| IBIS file for GS8662xxxBD
| Package: standard 165pin BGA
| DQ driver is programmable
| VDD 1.8V, VDDQ 1.5V or 1.8V
| Date:
| Rev 1.1 11/12/10 1) Pin F10 on Q36 pacakge changed from DIN to PROGBUF
[IBIS Ver]   4.2
[File name]   8662xxxbd.ibs
[File Rev]   1.1
[Date]   11/12/10
[Component]   GS8662D08BD
[Manufacturer]   GSI Technology
[Package]
|  variable   typ   min   max
R_pkg   0.2   0.1   0.5
L_pkg   3nH   1nH   5nH
C_pkg   1.5pF   1pF   3pF
[Package Model]   8662xxxBD
[Pin Mapping] pulldown_ref pullup_ref gnd_clamp_ref power_clamp_ref ext_ref
|PIN   Pull-Down   Pull-Up   Power-clamp   Gnd-clamp   EXT-ref
 A1   VSS   VDDQ   VSS   VDD
 A2   NC   NC   VSS   VDD   VREF
 A3   NC   NC   VSS   VDD   VREF
 A4   NC   NC   VSS   VDD   VREF
 A5   NC   NC   VSS   VDD   VREF
 A6   NC   NC   VSS   VDD   VREF
 A7   NC   NC   VSS   VDD   VREF
 A8   NC   NC   VSS   VDD   VREF
 A9   NC   NC   VSS   VDD   VREF
 A10   NC   NC   VSS   VDD   VREF
 A11   VSS   VDDQ   VSS   VDD
 B1   NC   NC
 B2   NC   NC
 B3   NC   NC
 B4   NC   NC   VSS   VDD   VREF
 B5   NC   NC
 B6   NC   NC   VSS   VDD   VREF
 B7   NC   NC   VSS   VDD   VREF
 B8   NC   NC   VSS   VDD   VREF
 B9   NC   NC
 B10   NC   NC
 B11   VSS   VDDQ   VSS   VDD
 C1   NC   NC
 C2   NC   NC
 C3   NC   NC
 C4   VSS   NC
 C5   NC   NC   VSS   VDD   VREF
 C6   NC   NC
 C7   NC   NC   VSS   VDD   VREF
 C8   VSS   NC
 C9   NC   NC
C10   NC   NC
 C11   NC   NC   VSS   VDD   VREF
 D1   NC   NC
 D2   NC   NC   VSS   VDD   VREF
 D3   NC   NC
 D4   VSS   NC
 D5   VSS   NC
 D6   VSS   NC
 D7   VSS   NC
 D8   VSS   NC
 D9   NC   NC
 D10   NC   NC
 D11   NC   NC
 E1   NC   NC
 E2   NC   NC
 E3   NC   NC
 E4   NC   VDDQ
 E5   VSS   NC
 E6   VSS   NC
 E7   VSS   NC
 E8   NC   VDDQ
 E9   NC   NC
 E10   NC   NC   VSS   VDD   VREF
 E11   VSS   VDDQ   VSS   VDD
 F1   NC   NC
 F2   NC   NC
 F3   NC   NC
 F4   NC   VDDQ
 F5   NC   VDD
 F6   VSS   NC
 F7   NC   VDD
 F8   NC   VDDQ
 F9   NC   NC
 F10   NC   NC
 F11   NC   NC
 G1   NC   NC
 G2   NC   NC   VSS   VDD   VREF
 G3   VSS   VDDQ   VSS   VDD
 G4   NC   VDDQ
 G5   NC   VDD
 G6   VSS   NC
 G7   NC   VDD
 G8   NC   VDDQ
 G9   NC   NC
 G10   NC   NC
 G11   NC   NC
 H1   NC   NC   VSS   VDD   VREF
 H2   NC   VREF
 H3   NC   VDDQ
 H4   NC   VDDQ
 H5   NC   VDD
 H6   VSS   NC
 H7   NC   VDD
 H8   NC   VDDQ
 H9   NC   VDDQ
 H10   NC   VREF
 H11   NC   NC
 J1   NC   NC
 J2   NC   NC
 J3   NC   NC
 J4   NC   VDDQ
 J5   NC   VDD
 J6   VSS   NC
 J7   NC   VDD
 J8   NC   VDDQ
 J9   NC   NC
 J10   VSS   VDDQ   VSS   VDD
 J11   NC   NC   VSS   VDD   VREF
 K1   NC   NC
 K2   NC   NC
 K3   NC   NC
 K4   NC   VDDQ
 K5   NC   VDD
 K6   VSS   NC
 K7   NC   VDD
 K8   NC   VDDQ
 K9   NC   NC
 K10   NC   NC
 K11   NC   NC
 L1   NC   NC
 L2   VSS   VDDQ   VSS   VDD
 L3   NC   NC   VSS   VDD   VREF
 L4   NC   VDDQ
 L5   VSS   NC
 L6   VSS   NC
 L7   VSS   NC
 L8   NC   VDDQ
 L9   NC   NC
 L10   NC   NC
 L11   VSS   VDDQ   VSS   VDD
 M1   NC   NC
 M2   NC   NC
 M3   NC   NC
 M4   VSS   NC
 M5   VSS   NC
 M6   VSS   NC
 M7   VSS   NC
 M8   VSS   NC
 M9   NC   NC
 M10   NC   NC
 M11   NC   NC   VSS   VDD   VREF
 N1   NC   NC
 N2   NC   NC   VSS   VDD   VREF
 N3   NC   NC
 N4   VSS   NC
 N5   NC   NC   VSS   VDD   VREF
 N6   NC   NC   VSS   VDD   VREF
 N7   NC   NC   VSS   VDD   VREF
 N8   VSS   NC
 N9   NC   NC
 N10   NC   NC
 N11   NC   NC
 P1   NC   NC
 P2   NC   NC
 P3   VSS   VDDQ   VSS   VDD
 P4   NC   NC   VSS   VDD   VREF
 P5   NC   NC   VSS   VDD   VREF
 P6   NC   NC   VSS   VDD   VREF
 P7   NC   NC   VSS   VDD   VREF
 P8   NC   NC   VSS   VDD   VREF
 P9   NC   NC
 P10   NC   NC
 P11   NC   NC
 R1   VSS   VDDQ   VSS   VDD
 R2   NC   NC   VSS   VDD   VREF
 R3   NC   NC   VSS   VDD   VREF
 R4   NC   NC   VSS   VDD   VREF
 R5   NC   NC   VSS   VDD   VREF
 R6   NC   NC   VSS   VDD   VREF
 R7   NC   NC   VSS   VDD   VREF
 R8   NC   NC   VSS   VDD   VREF
 R9   NC   NC   VSS   VDD   VREF
 R10   NC   NC   VSS   VDD   VREF
 R11   NC   NC   VSS   VDD   VREF
[Pin]   signal_name model_name   R_pin   L_pin   C_pin
 A1   nCQ   ECHO   229m   1.82nH   0.656pF
 A2   SA   CONTROL   203m   1.74nH   0.634pF
 A3   SA   CONTROL   185m   1.59nH   0.518pF
 A4   nW   CONTROL   185m   1.38nH   0.583pF
 A5   nNW1   CONTROL   178m   1.36nH   0.540pF
 A6   nK   CONTROL   224m   1.64nH   0.652pF
 A7   SA   CONTROL   185m   1.39nH   0.547pF
 A8   nR   CONTROL   188m   1.49nH   0.551pF
 A9   SA   CONTROL   186m   1.48nH   0.595pF
 A10   SA   CONTROL   191m   1.70nH   0.568pF
 A11   CQ   ECHO   227m   1.84nH   0.605pF
 B1   NC   NC
 B2   NC   NC
 B3   NC   NC
 B4   SA   CONTROL   181m   1.49nH   0.521pF
 B5   NC   NC
 B6   K   CONTROL   221m   1.68nH   0.652pF
 B7   nNW0   CONTROL   178m   1.43nH   0.537pF
 B8   SA   CONTROL   181m   1.41nH   0.565pF
 B9   NC   NC
 B10   NC   NC
 B11   Q3   PROGBUF   232m   1.94nH   0.683pF
 C1   NC   NC
 C2   NC   NC
 C3   NC   NC
 C4   VSS   GND
 C5   SA   CONTROL   189m   1.61nH   0.614pF
 C6   NC   NC
 C7   SA   CONTROL   185m   1.72nH   0.535pF
 C8   VSS   GND
 C9   NC   NC
 C10   NC   NC
 C11   D3   DIN   219m   1.74nH   0.625pF
 D1   NC   NC
 D2   D4   DIN   227m   1.95nH   0.654pF
 D3   NC   NC
 D4   VSS   GND
 D5   VSS   GND
 D6   VSS   GND
 D7   VSS   GND
 D8   VSS   GND
 D9   NC   NC
 D10   NC   NC
 D11   Nc   NC
 E1   Nc   NC
 E2   Nc   NC
 E3   Q4   PROGBUF   240m   2.04nH   0.712pF
 E4   VDDQ   POWER
 E5   VSS   GND
 E6   VSS   GND
 E7   VSS   GND
 E8   VDDQ   POWER
 E9   NC   NC
 E10   D2   DIN   223m   1.85nH   0.659pF
 E11   Q2   PROGBUF   225m   1.74nH   0.649pF
 F1   NC   NC
 F2   NC   NC
 F3   NC   NC
 F4   VDDQ   POWER
 F5   VDD   POWER
 F6   VSS   GND
 F7   VDD   POWER
 F8   VDDQ   POWER
 F9   NC   NC
 F10   NC   NC
 F11   NC   NC
 G1   NC   NC
 G2   D5   DIN   221m   1.73nH   0.669pF
 G3   Q5   PROGBUF   244m   2.11nH   0.723pF
 G4   VDDQ   POWER
 G5   VDD   POWER
 G6   VSS   GND
 G7   VDD   POWER
 G8   VDDQ   POWER
 G9   NC   NC
 G10   NC   NC
 G11   NC   NC
 H1   NDoff   CONTROL   254m   2.26nH   0.651pF
 H2   VREF   POWER
 H3   VDDQ   POWER
 H4   VDDQ   POWER
 H5   VDD   POWER
 H6   VSS   GND
 H7   VDD   POWER
 H8   VDDQ   POWER
 H9   VDDQ   POWER
 H10   VREF   POWER
 H11   ZQ   NC
 J1   NC   NC
 J2   NC   NC
 J3   NC   NC
 J4   VDDQ   POWER
 J5   VDD   POWER
 J6   VSS   GND
 J7   VDD   POWER
 J8   VDDQ   POWER
 J9   NC   NC
 J10   Q1   PROGBUF   231m   1.92nH   0.628pF
 J11   D1   DIN   222m   1.68nH   0.657pF
 K1   NC   NC
 K2   NC   NC
 K3   NC   NC
 K4   VDDQ   POWER
 K5   VDD   POWER
 K6   VSS   GND
 K7   VDD   POWER
 K8   VDDQ   POWER
 K9   NC   NC
 K10   NC   NC
 K11   NC   NC
 L1   NC   NC
 L2   Q6   PROGBUF   228m   1.89nH   0.672pF
 L3   D6   DIN   237m   2.14nH   0.663pF
 L4   VDDQ   POWER
 L5   VSS   GND
 L6   VSS   GND
 L7   VSS   GND
 L8   VDDQ   POWER
 L9   NC   NC
 L10   NC   NC
 L11   Q0   PROGBUF   223m   1.72nH   0.654pF
 M1   NC   NC
 M2   NC   NC
 M3   NC   NC
 M4   VSS   GND
 M5   VSS   GND
 M6   VSS   GND
 M7   VSS   GND
 M8   VSS   GND
 M9   NC   NC
 M10   NC   NC
 M11   D0   DIN   228m   1.90nH   0.609pF
 N1   NC   NC
 N2   D7   DIN   219m   1.88nH   0.569pF
 N3   NC   NC
 N4   VSS   GND
 N5   SA   CONTROL   186m   1.69nH   0.505pF
 N6   SA   CONTROL   191m   1.56nH   0.607pF
 N7   SA   CONTROL   193m   1.62nH   0.543pF
 N8   VSS   GND
 N9   NC   NC
 N10   NC   NC
 N11   NC   NC
 P1   NC   NC
 P2   NC   NC
 P3   Q7   PROGBUF   236m   2.33nH   0.676pF
 P4   SA   CONTROL   185m   1.52nH   0.546pF
 P5   SA   CONTROL   185m   1.41nH   0.604pF
 P6   C   CONTROL   184m   1.42nH   0.590pF
 P7   SA   CONTROL   192m   1.57nH   0.599pF
 P8   SA   CONTROL   195m   1.51nH   0.593pF
 P9   NC   NC
 P10   NC   NC
 P11   NC   NC
 R1   TDO   JTAG   151m   1.27nH   0.509pF
 R2   TCK   CONTROL   132m   1.10nH   0.478pF
 R3   SA   CONTROL   208m   1.92nH   0.490pF
 R4   SA   CONTROL   198m   1.58nH   0.599pF
 R5   SA   CONTROL   190m   1.46nH   0.609pF
 R6   CBar   CONTROL   196m   1.46nH   0.608pF
 R7   SA   CONTROL   198m   1.47nH   0.632pF
 R8   SA   CONTROL   202m   1.49nH   0.640pF
 R9   SA   CONTROL   214m   1.68nH   0.647pF
 R10   TMS   CONTROL   148m   1.19nH   0.517pF
 R11   TDI   CONTROL   157m   1.27nH   0.525pF
[Component]   GS8662D09BD
[Manufacturer]   GSI Technology
[Package]
|  variable   typ   min   max
R_pkg   0.2   0.1   0.5
L_pkg   3nH   1nH   5nH
C_pkg   1.5pF   1pF   3pF
[Package Model]   8662xxxBD
[Pin Mapping] pulldown_ref pullup_ref gnd_clamp_ref power_clamp_ref ext_ref
|PIN   Pull-Down   Pull-Up   Power-clamp   Gnd-clamp   EXT-ref
 A1   VSS   VDDQ   VSS   VDD
 A2   NC   NC   VSS   VDD   VREF
 A3   NC   NC   VSS   VDD   VREF
 A4   NC   NC   VSS   VDD   VREF
 A5   NC   NC   VSS   VDD   VREF
 A6   NC   NC   VSS   VDD   VREF
 A7   NC   NC   VSS   VDD   VREF
 A8   NC   NC   VSS   VDD   VREF
 A9   NC   NC   VSS   VDD   VREF
 A10   NC   NC   VSS   VDD   VREF
 A11   VSS   VDDQ   VSS   VDD
 B1   NC   NC
 B2   NC   NC
 B3   NC   NC
 B4   NC   NC   VSS   VDD   VREF
 B5   NC   NC
 B6   NC   NC   VSS   VDD   VREF
 B7   NC   NC   VSS   VDD   VREF
 B8   NC   NC   VSS   VDD   VREF
 B9   NC   NC
 B10   NC   NC
 B11   VSS   VDDQ   VSS   VDD
 C1   NC   NC
 C2   NC   NC
 C3   NC   NC
 C4   VSS   NC
 C5   NC   NC   VSS   VDD   VREF
 C6   NC   NC
 C7   NC   NC   VSS   VDD   VREF
 C8   VSS   NC
 C9   NC   NC
 C10   NC   NC
 C11   NC   NC   VSS   VDD   VREF
 D1   NC   NC
 D2   NC   NC   VSS   VDD   VREF
 D3   NC   NC
 D4   VSS   NC
 D5   VSS   NC
 D6   VSS   NC
 D7   VSS   NC
 D8   VSS   NC
 D9   NC   NC
 D10   NC   NC
 D11   NC   NC
 E1   NC   NC
 E2   NC   NC
 E3   VSS   VDDQ   VSS   VDD
 E4   NC   VDDQ
 E5   VSS   NC
 E6   VSS   NC
 E7   VSS   NC
 E8   NC   VDDQ
 E9   NC   NC
 E10   NC   NC   VSS   VDD   VREF
 E11   VSS   VDDQ   VSS   VDD
 F1   NC   NC
 F2   NC   NC
 F3   NC   NC
 F4   NC   VDDQ
 F5   NC   VDD
 F6   VSS   NC
 F7   NC   VDD
 F8   NC   VDDQ
 F9   NC   NC
 F10   NC   NC
 F11   NC   NC
 G1   NC   NC
 G2   NC   NC   VSS   VDD   VREF
 G3   VSS   VDDQ   VSS   VDD
 G4   NC   VDDQ
 G5   NC   VDD
 G6   VSS   NC
 G7   NC   VDD
 G8   NC   VDDQ
 G9   NC   NC
 G10   NC   NC
 G11   NC   NC
 H1   NC   NC   VSS   VDD   VREF
 H2   NC   VREF
 H3   NC   VDDQ
 H4   NC   VDDQ
 H5   NC   VDD
 H6   VSS   NC
 H7   NC   VDD
 H8   NC   VDDQ
 H9   NC   VDDQ
 H10   NC   VREF
 H11   NC   NC
 J1   NC   NC
 J2   NC   NC
 J3   NC   NC
 J4   NC   VDDQ
 J5   NC   VDD
 J6   VSS   NC
 J7   NC   VDD
 J8   NC   VDDQ
 J9   NC   NC
 J10   VSS   VDDQ   VSS   VDD
 J11   NC   NC   VSS   VDD   VREF
 K1   NC   NC
 K2   NC   NC
 K3   NC   NC
 K4   NC   VDDQ
 K5   NC   VDD
 K6   VSS   NC
 K7   NC   VDD
 K8   NC   VDDQ
 K9   NC   NC
 K10   NC   NC
 K11   NC   NC
 L1   NC   NC
 L2   VSS   VDDQ   VSS   VDD
 L3   NC   NC   VSS   VDD   VREF
 L4   NC   VDDQ
 L5   VSS   NC
 L6   VSS   NC
 L7   VSS   NC
 L8   NC   VDDQ
 L9   NC   NC
 L10   NC   NC
 L11   VSS   VDDQ   VSS   VDD
 M1   NC   NC
 M2   NC   NC
 M3   NC   NC
 M4   VSS   NC
 M5   VSS   NC
 M6   VSS   NC
 M7   VSS   NC
 M8   VSS   NC
 M9   NC   NC
 M10   NC   NC
 M11   NC   NC   VSS   VDD   VREF
 N1   NC   NC
 N2   NC   NC   VSS   VDD   VREF
 N3   NC   NC
 N4   VSS   NC
 N5   NC   NC   VSS   VDD   VREF
 N6   NC   NC   VSS   VDD   VREF
 N7   NC   NC   VSS   VDD   VREF
 N8   VSS   NC
 N9   NC   NC
 N10   NC   NC
 N11   NC   NC
 P1   NC   NC
 P2   NC   NC
 P3   VSS   VDDQ   VSS   VDD
 P4   NC   NC   VSS   VDD   VREF
 P5   NC   NC   VSS   VDD   VREF
 P6   NC   NC   VSS   VDD   VREF
 P7   NC   NC   VSS   VDD   VREF
 P8   NC   NC   VSS   VDD   VREF
 P9   NC   NC
 P10   NC   NC   VSS   VDD   VREF
 P11   VSS   VDDQ   VSS   VDD
 R1   VSS   VDDQ   VSS   VDD
 R2   NC   NC   VSS   VDD   VREF
 R3   NC   NC   VSS   VDD   VREF
 R4   NC   NC   VSS   VDD   VREF
 R5   NC   NC   VSS   VDD   VREF
 R6   NC   NC   VSS   VDD   VREF
 R7   NC   NC   VSS   VDD   VREF
 R8   NC   NC   VSS   VDD   VREF
 R9   NC   NC   VSS   VDD   VREF
 R10   NC   NC   VSS   VDD   VREF
 R11   NC   NC   VSS   VDD   VREF
[Pin]   signal_name model_name   R_pin   L_pin   C_pin
 A1   nCQ   ECHO   229m   1.82nH   0.656pF
 A2   SA   CONTROL   203m   1.74nH   0.634pF
 A3   SA   CONTROL   185m   1.59nH   0.518pF
 A4   nW   CONTROL   185m   1.38nH   0.583pF
 A5   nBW1   CONTROL   178m   1.36nH   0.540pF
 A6   nK   CONTROL   224m   1.64nH   0.652pF
 A7   SA   CONTROL   185m   1.39nH   0.547pF
 A8   nR   CONTROL   188m   1.49nH   0.551pF
 A9   SA   CONTROL   186m   1.48nH   0.595pF
 A10   SA   CONTROL   191m   1.70nH   0.568pF
 A11   CQ   ECHO   227m   1.84nH   0.605pF
 B1   NC   NC
 B2   NC   NC
 B3   NC   NC
 B4   SA   CONTROL   181m   1.49nH   0.521pF
 B5   NC   NC
 B6   K   CONTROL   221m   1.68nH   0.652pF
 B7   NBW0   CONTROL   178m   1.43nH   0.537pF
 B8   SA   CONTROL   181m   1.41nH   0.565pF
 B9   NC   NC
 B10   NC   NC
 B11   Q4   PROGBUF   232m   1.94nH   0.683pF
 C1   NC   NC
 C2   NC   NC
 C3   NC   NC
 C4   VSS   GND
 C5   SA   CONTROL   189m   1.61nH   0.614pF
 C6   NC   NC
 C7   SA   CONTROL   185m   1.72nH   0.535pF
 C8   VSS   GND
 C9   NC   NC
 C10   NC   NC
 C11   D4   DIN   219m   1.74nH   0.625pF
 D1   NC   NC
 D2   D5   DIN   227m   1.95nH   0.654pF
 D3   NC   NC
 D4   VSS   GND
 D5   VSS   GND
 D6   VSS   GND
 D7   VSS   GND
 D8   VSS   GND
 D9   NC   NC
 D10   NC   NC
 D11   NC   NC
 E1   NC   NC
 E2   NC   NC
 E3   Q5   PROGBUF   240m   2.04nH   0.712pF
 E4   VDDQ   POWER
 E5   VSS   GND
 E6   VSS   GND
 E7   VSS   GND
 E8   VDDQ   POWER
 E9   NC   NC
 E10   D3   DIN   223m   1.85nH   0.659pF
 E11   Q3   PROGBUF   225m   1.74nH   0.649pF
 F1   NC   NC
 F2   NC   NC
 F3   NC   NC
 F4   VDDQ   POWER
 F5   VDD   POWER
 F6   VSS   GND
 F7   VDD   POWER
 F8   VDDQ   POWER
 F9   NC   NC
 F10   NC   NC
 F11   NC   NC
 G1   NC   NC
 G2   D6   DIN   221m   1.73nH   0.669pF
 G3   Q6   PROGBUF   244m   2.11nH   0.723pF
 G4   VDDQ   POWER
 G5   VDD   POWER
 G6   VSS   GND
 G7   VDD   POWER
 G8   VDDQ   POWER
 G9   NC   NC
 G10   NC   NC
 G11   NC   NC
 H1   NDoff   CONTROL   254m   2.26nH   0.651pF
 H2   VREF   POWER
 H3   VDDQ   POWER
 H4   VDDQ   POWER
 H5   VDD   POWER
 H6   VSS   GND
 H7   VDD   POWER
 H8   VDDQ   POWER
 H9   VDDQ   POWER
 H10   VREF   POWER
 H11   ZQ   NC
 J1   NC   NC
 J2   NC   NC
 J3   NC   NC
 J4   VDDQ   POWER
 J5   VDD   POWER
 J6   VSS   GND
 J7   VDD   POWER
 J8   VDDQ   POWER
 J9   NC   NC
 J10   Q2   PROGBUF   231m   1.92nH   0.628pF
 J11   D2   DIN   222m   1.68nH   0.657pF
 K1   NC   NC
 K2   NC   NC
 K3   NC   NC
 K4   VDDQ   POWER
 K5   VDD   POWER
 K6   VSS   GND
 K7   VDD   POWER
 K8   VDDQ   POWER
 K9   NC   NC
 K10   NC   NC
 K11   NC   NC
 L1   NC   NC
 L2   Q7   PROGBUF   228m   1.89nH   0.672pF
 L3   D7   DIN   237m   2.14nH   0.663pF
 L4   VDDQ   POWER
 L5   VSS   GND
 L6   VSS   GND
 L7   VSS   GND
 L8   VDDQ   POWER
 L9   NC   NC
 L10   NC   NC
 L11   Q1   PROGBUF   223m   1.72nH   0.654pF
 M1   NC   NC
 M2   NC   NC
 M3   NC   NC
 M4   VSS   GND
 M5   VSS   GND
 M6   VSS   GND
 M7   VSS   GND
 M8   VSS   GND
 M9   NC   NC
 M10   NC   NC
 M11   D1   DIN   228m   1.90nH   0.609pF
 N1   NC   NC
 N2   D8   DIN   219m   1.88nH   0.569pF
 N3   NC   NC
 N4   VSS   GND
 N5   SA   CONTROL   186m   1.69nH   0.505pF
 N6   SA   CONTROL   191m   1.56nH   0.607pF
 N7   SA   CONTROL   193m   1.62nH   0.543pF
 N8   VSS   GND
 N9   NC   NC
 N10   NC   NC
 N11   NC   NC
 P1   NC   NC
 P2   NC   NC
 P3   Q8   PROGBUF   236m   2.33nH   0.676pF
 P4   SA   CONTROL   185m   1.52nH   0.546pF
 P5   SA   CONTROL   185m   1.41nH   0.604pF
 P6   C   CONTROL   184m   1.42nH   0.590pF
 P7   SA   CONTROL   192m   1.57nH   0.599pF
 P8   SA   CONTROL   195m   1.51nH   0.593pF
 P9   NC   NC
 P10   D0   DIN   221m   1.90nH   0.660pF
 P11   Q0   PROGBUF   236m   1.77nH   0.674pF
 R1   TDO   JTAG   151m   1.27nH   0.509pF
 R2   TCK   CONTROL   132m   1.10nH   0.478pF
 R3   SA   CONTROL   208m   1.92nH   0.490pF
 R4   SA   CONTROL   198m   1.58nH   0.599pF
 R5   SA   CONTROL   190m   1.46nH   0.609pF
 R6   CBar   CONTROL   196m   1.46nH   0.608pF
 R7   SA   CONTROL   198m   1.47nH   0.632pF
 R8   SA   CONTROL   202m   1.49nH   0.640pF
 R9   SA   CONTROL   214m   1.68nH   0.647pF
 R10   TMS   CONTROL   148m   1.19nH   0.517pF
 R11   TDI   CONTROL   157m   1.27nH   0.525pF
[Component]   GS8662D18BD
[Manufacturer]   GSI Technology
[Package]
|  variable   typ   min   max
R_pkg   0.2   0.1   0.5
L_pkg   3nH   1nH   5nH
C_pkg   1.5pF   1pF   3pF
[Package Model]   8662xxxBD
[Pin Mapping] pulldown_ref pullup_ref gnd_clamp_ref power_clamp_ref ext_ref
|PIN   Pull-Down   Pull-Up   Power-clamp   Gnd-clamp   EXT-ref
 A1   VSS   VDDQ   VSS   VDD
 A2   NC   NC   VSS   VDD   VREF
 A3   NC   NC   VSS   VDD   VREF
 A4   NC   NC   VSS   VDD   VREF
 A5   NC   NC   VSS   VDD   VREF
 A6   NC   NC   VSS   VDD   VREF
 A7   NC   NC
 A8   NC   NC   VSS   VDD   VREF
 A9   NC   NC   VSS   VDD   VREF
 A10   NC   NC   VSS   VDD   VREF
 A11   VSS   VDDQ   VSS   VDD
 B1   NC   NC
 B2   VSS   VDDQ   VSS   VDD
 B3   NC   NC   VSS   VDD   VREF
 B4   NC   NC   VSS   VDD   VREF
 B5   NC   NC
 B6   NC   NC   VSS   VDD   VREF
 B7   NC   NC   VSS   VDD   VREF
 B8   NC   NC   VSS   VDD   VREF
 B9   NC   NC
 B10   NC   NC
 B11   VSS   VDDQ   VSS   VDD
 C1   NC   NC
 C2   NC   NC
 C3   NC   NC   VSS   VDD   VREF
 C4   VSS   NC
 C5   NC   NC   VSS   VDD   VREF
 C6   NC   NC
 C7   NC   NC   VSS   VDD   VREF
 C8   VSS   NC
 C9   NC   NC
 C10   VSS   VDDQ   VSS   VDD
 C11   NC   NC   VSS   VDD   VREF
 D1   NC   NC
 D2   NC   NC   VSS   VDD   VREF
 D3   VSS   VDDQ   VSS   VDD
 D4   VSS   NC
 D5   VSS   NC
 D6   VSS   NC
 D7   VSS   NC
 D8   VSS   NC
 D9   NC   NC
 D10   NC   NC
 D11   NC   NC   VSS   VDD   VREF
 E1   NC   NC
 E2   NC   NC
 E3   VSS   VDDQ   VSS   VDD
 E4   NC   VDDQ
 E5   VSS   NC
 E6   VSS   NC
 E7   VSS   NC
 E8   NC   VDDQ
 E9   NC   NC
 E10   NC   NC   VSS   VDD   VREF
 E11   VSS   VDDQ   VSS   VDD
 F1   NC   NC
 F2   VSS   VDDQ   VSS   VDD
 F3   NC   NC   VSS   VDD   VREF
 F4   NC   VDDQ
 F5   NC   VDD
 F6   VSS   NC
 F7   NC   VDD
 F8   NC   VDDQ
 F9   NC   NC
 F10   NC   NC
 F11   VSS   VDDQ   VSS   VDD
 G1   NC   NC
 G2   NC   NC   VSS   VDD   VREF
 G3   VSS   VDDQ   VSS   VDD
 G4   NC   VDDQ
 G5   NC   VDD
 G6   VSS   NC
 G7   NC   VDD
 G8   NC   VDDQ
 G9   NC   NC
 G10   NC   NC
 G11   NC   NC   VSS   VDD   VREF
 H1   NC   NC   VSS   VDD   VREF
 H2   NC   VREF
 H3   NC   VDDQ
 H4   NC   VDDQ
 H5   NC   VDD
 H6   VSS   NC
 H7   NC   VDD
 H8   NC   VDDQ
 H9   NC   VDDQ
 H10   NC   VREF
 H11   NC   NC
 J1   NC   NC
 J2   NC   NC
 J3   NC   NC   VSS   VDD   VREF
 J4   NC   VDDQ
 J5   NC   VDD
 J6   VSS   NC
 J7   NC   VDD
 J8   NC   VDDQ
 J9   NC   NC
 J10   VSS   VDDQ   VSS   VDD
 J11   NC   NC   VSS   VDD   VREF
 K1   NC   NC
 K2   NC   NC
 K3   VSS   VDDQ   VSS   VDD
 K4   NC   VDDQ
 K5   NC   VDD
 K6   VSS   NC
 K7   NC   VDD
 K8   NC   VDDQ
 K9   NC   NC
 K10   NC   NC   VSS   VDD   VREF
 K11   VSS   VDDQ   VSS   VDD
 L1   NC   NC
 L2   VSS   VDDQ   VSS   VDD
 L3   NC   NC   VSS   VDD   VREF
 L4   NC   VDDQ
 L5   VSS   NC
 L6   VSS   NC
 L7   VSS   NC
 L8   NC   VDDQ
 L9   NC   NC
 L10   NC   NC
 L11   VSS   VDDQ   VSS   VDD
 M1   NC   NC
 M2   NC   NC
 M3   NC   NC   VSS   VDD   VREF
 M4   VSS   NC
 M5   VSS   NC
 M6   VSS   NC
 M7   VSS   NC
 M8   VSS   NC
 M9   NC   NC
 M10   VSS   VDDQ   VSS   VDD
 M11   NC   NC   VSS   VDD   VREF
 N1   NC   NC
 N2   NC   NC   VSS   VDD   VREF
 N3   VSS   VDDQ   VSS   VDD
 N4   VSS   NC
 N5   NC   NC   VSS   VDD   VREF
 N6   NC   NC   VSS   VDD   VREF
 N7   NC   NC   VSS   VDD   VREF
 N8   VSS   NC
 N9   NC   NC
 N10   NC   NC
 N11   NC   NC   VSS   VDD   VREF
 P1   NC   NC
 P2   NC   NC
 P3   VSS   VDDQ   VSS   VDD
 P4   NC   NC   VSS   VDD   VREF
 P5   NC   NC   VSS   VDD   VREF
 P6   NC   NC   VSS   VDD   VREF
 P7   NC   NC   VSS   VDD   VREF
 P8   NC   NC   VSS   VDD   VREF
 P9   NC   NC
 P10   NC   NC   VSS   VDD   VREF
 P11   VSS   VDDQ   VSS   VDD
 R1   VSS   VDDQ   VSS   VDD
 R2   NC   NC   VSS   VDD   VREF
 R3   NC   NC   VSS   VDD   VREF
 R4   NC   NC   VSS   VDD   VREF
 R5   NC   NC   VSS   VDD   VREF
 R6   NC   NC   VSS   VDD   VREF
 R7   NC   NC   VSS   VDD   VREF
 R8   NC   NC   VSS   VDD   VREF
 R9   NC   NC   VSS   VDD   VREF
 R10   NC   NC   VSS   VDD   VREF
 R11   NC   NC   VSS   VDD   VREF
[Pin]   signal_name model_name   R_pin   L_pin   C_pin
 A1   nCQ   ECHO   229m   1.82nH   0.656pF
 A2   SA   CONTROL   203m   1.74nH   0.634pF
 A3   SA   CONTROL   185m   1.59nH   0.518pF
 A4   nW   CONTROL   185m   1.38nH   0.583pF
 A5   nBW1   CONTROL   178m   1.36nH   0.540pF
 A6   nK   CONTROL   224m   1.64nH   0.652pF
 A7   NC   NC
 A8   nR   CONTROL   188m   1.49nH   0.551pF
 A9   SA   CONTROL   186m   1.48nH   0.595pF
 A10   SA   CONTROL   191m   1.70nH   0.568pF
 A11   CQ   ECHO   227m   1.84nH   0.605pF
 B1   NC   NC
 B2   Q9   PROGBUF   233m   1.94nH   0.666pF
 B3   D9   DIN   226m   2.49nH   0.560pF
 B4   SA   CONTROL   181m   1.49nH   0.521pF
 B5   NC   NC
 B6   K   CONTROL   221m   1.68nH   0.652pF
 B7   NBW0   CONTROL   178m   1.43nH   0.537pF
 B8   SA   CONTROL   181m   1.41nH   0.565pF
 B9   NC   NC
 B10   NC   NC
 B11   Q8   PROGBUF   232m   1.94nH   0.683pF
 C1   NC   NC
 C2   NC   NC
 C3   D10   DIN   241m   2.35nH   0.708pF
 C4   VSS   GND
 C5   SA   CONTROL   189m   1.61nH   0.614pF
 C6   NC   NC
 C7   SA   CONTROL   185m   1.72nH   0.535pF
 C8   VSS   GND
 C9   NC   NC
 C10   Q7   PROGBUF   231m   2.16nH   0.604pF
 C11   D8   DIN   219m   1.74nH   0.625pF
 D1   NC   NC
 D2   D11   DIN   227m   1.95nH   0.654pF
 D3   Q10   PROGBUF   256m   2.33nH   0.752pF
 D4   VSS   GND
 D5   VSS   GND
 D6   VSS   GND
 D7   VSS   GND
 D8   VSS   GND
 D9   NC   NC
 D10   NC   NC
 D11   D7   DIN   218m   1.75nH   0.605pF
 E1   NC   NC
 E2   NC   NC
 E3   Q11   PROGBUF   240m   2.04nH   0.712pF
 E4   VDDQ   POWER
 E5   VSS   GND
 E6   VSS   GND
 E7   VSS   GND
 E8   VDDQ   POWER
 E9   NC   NC
 E10   D6   DIN   223m   1.85nH   0.659pF
 E11   Q6   PROGBUF   225m   1.74nH   0.649pF
 F1   NC   NC
 F2   Q12   PROGBUF   230m   1.84nH   0.651pF
 F3   D12   DIN   230m   2.00nH   0.644pF
 F4   VDDQ   POWER
 F5   VDD   POWER
 F6   VSS   GND
 F7   VDD   POWER
 F8   VDDQ   POWER
 F9   NC   NC
 F10   NC   NC
 F11   Q5   PROGBUF   237m   1.82nH   0.690pF
 G1   NC   NC
 G2   D13   DIN   221m   1.73nH   0.669pF
 G3   Q13   PROGBUF   244m   2.11nH   0.723pF
 G4   VDDQ   POWER
 G5   VDD   POWER
 G6   VSS   GND
 G7   VDD   POWER
 G8   VDDQ   POWER
 G9   NC   NC
 G10   NC   NC
 G11   D5   DIN   217m   1.66nH   0.597pF
 H1   NDoff   CONTROL   254m   2.26nH   0.651pF
 H2   VREF   POWER
 H3   VDDQ   POWER
 H4   VDDQ   POWER
 H5   VDD   POWER
 H6   VSS   GND
 H7   VDD   POWER
 H8   VDDQ   POWER
 H9   VDDQ   POWER
 H10   VREF   POWER
 H11   ZQ   NC
 J1   NC   NC
 J2   NC   NC
 J3   D14   DIN   233m   2.02nH   0.708pF
 J4   VDDQ   POWER
 J5   VDD   POWER
 J6   VSS   GND
 J7   VDD   POWER
 J8   VDDQ   POWER
 J9   NC   NC
 J10   Q4   PROGBUF   231m   1.92nH   0.628pF
 J11   D4   DIN   222m   1.68nH   0.657pF
 K1   NC   NC
 K2   NC   NC
 K3   Q14   PROGBUF   238m   1.99nH   0.619pF
 K4   VDDQ   POWER
 K5   VDD   POWER
 K6   VSS   GND
 K7   VDD   POWER
 K8   VDDQ   POWER
 K9   NC   NC
 K10   D3   DIN   211m   1.71nH   0.543pF
 K11   Q3   PROGBUF   236m   1.79nH   0.629pF
 L1   NC   NC
 L2   Q15   PROGBUF   228m   1.89nH   0.672pF
 L3   D15   DIN   237m   2.14nH   0.663pF
 L4   VDDQ   POWER
 L5   VSS   GND
 L6   VSS   GND
 L7   VSS   GND
 L8   VDDQ   POWER
 L9   NC   NC
 L10   NC   NC
 L11   Q2   PROGBUF   223m   1.72nH   0.654pF
 M1   NC   NC
 M2   NC   NC
 M3   D16   DIN   246m   2.04nH   0.704pF
 M4   VSS   GND
 M5   VSS   GND
 M6   VSS   GND
 M7   VSS   GND
 M8   VSS   GND
 M9   NC   NC
 M10   Q1   PROGBUF   243m   2.05nH   0.690pF
 M11   D2   DIN   228m   1.90nH   0.609pF
 N1   NC   NC
 N2   D17   DIN   219m   1.88nH   0.569pF
 N3   Q16   PROGBUF   268m   2.36nH   0.730pF
 N4   VSS   GND
 N5   SA   CONTROL   186m   1.69nH   0.505pF
 N6   SA   CONTROL   191m   1.56nH   0.607pF
 N7   SA   CONTROL   193m   1.62nH   0.543pF
 N8   VSS   GND
 N9   NC   NC
 N10   NC   NC
 N11   D1   DIN   220m   1.66nH   0.645pF
 P1   NC   NC
 P2   NC   NC
 P3   Q17   PROGBUF   236m   2.33nH   0.676pF
 P4   SA   CONTROL   185m   1.52nH   0.546pF
 P5   SA   CONTROL   185m   1.41nH   0.604pF
 P6   C   CONTROL   184m   1.42nH   0.590pF
 P7   SA   CONTROL   192m   1.57nH   0.599pF
 P8   SA   CONTROL   195m   1.51nH   0.593pF
 P9   NC   NC
 P10   D0   DIN   221m   1.90nH   0.660pF
 P11   Q0   PROGBUF   236m   1.77nH   0.674pF
 R1   TDO   JTAG   151m   1.27nH   0.509pF
 R2   TCK   CONTROL   132m   1.10nH   0.478pF
 R3   SA   CONTROL   208m   1.92nH   0.490pF
 R4   SA   CONTROL   198m   1.58nH   0.599pF
 R5   SA   CONTROL   190m   1.46nH   0.609pF
 R6   CBar   CONTROL   196m   1.46nH   0.608pF
 R7   SA   CONTROL   198m   1.47nH   0.632pF
 R8   SA   CONTROL   202m   1.49nH   0.640pF
 R9   SA   CONTROL   214m   1.68nH   0.647pF
 R10   TMS   CONTROL   148m   1.19nH   0.517pF
 R11   TDI   CONTROL   157m   1.27nH   0.525pF
[Component]   GS8662D19BD
[Manufacturer]   GSI Technology
[Package]
|  variable   typ   min   max
R_pkg   0.2   0.1   0.5
L_pkg   3nH   1nH   5nH
C_pkg   1.5pF   1pF   3pF
[Package Model]   8662xxxBD
[Pin Mapping] pulldown_ref pullup_ref gnd_clamp_ref power_clamp_ref ext_ref
|PIN   Pull-Down   Pull-Up   Power-clamp   Gnd-clamp   EXT-ref
 A1   VSS   VDDQ   VSS   VDD
 A2   NC   NC   VSS   VDD   VREF
 A3   NC   NC   VSS   VDD   VREF
 A4   NC   NC   VSS   VDD   VREF
 A5   NC   NC   VSS   VDD   VREF
 A6   NC   NC   VSS   VDD   VREF
 A7   NC   NC
 A8   NC   NC   VSS   VDD   VREF
 A9   NC   NC   VSS   VDD   VREF
 A10   NC   NC   VSS   VDD   VREF
 A11   VSS   VDDQ   VSS   VDD
 B1   NC   NC
 B2   VSS   VDDQ   VSS   VDD
 B3   NC   NC   VSS   VDD   VREF
 B4   NC   NC   VSS   VDD   VREF
 B5   NC   NC
 B6   NC   NC   VSS   VDD   VREF
 B7   NC   NC   VSS   VDD   VREF
 B8   NC   NC   VSS   VDD   VREF
 B9   NC   NC
 B10   NC   NC
 B11   VSS   VDDQ   VSS   VDD
 C1   NC   NC
 C2   NC   NC
 C3   NC   NC   VSS   VDD   VREF
 C4   VSS   NC
 C5   NC   NC   VSS   VDD   VREF
 C6   NC   NC
 C7   NC   NC   VSS   VDD   VREF
 C8   VSS   NC
 C9   NC   NC
 C10   VSS   VDDQ   VSS   VDD
 C11   NC   NC   VSS   VDD   VREF
 D1   NC   NC
 D2   NC   NC   VSS   VDD   VREF
 D3   VSS   VDDQ   VSS   VDD
 D4   VSS   NC
 D5   VSS   NC
 D6   VSS   NC
 D7   VSS   NC
 D8   VSS   NC
 D9   NC   NC
 D10   NC   NC
 D11   NC   NC   VSS   VDD   VREF
 E1   NC   NC
 E2   NC   NC
 E3   VSS   VDDQ   VSS   VDD
 E4   NC   VDDQ
 E5   VSS   NC
 E6   VSS   NC
 E7   VSS   NC
 E8   NC   VDDQ
 E9   NC   NC
 E10   NC   NC   VSS   VDD   VREF
 E11   VSS   VDDQ   VSS   VDD
 F1   NC   NC
 F2   VSS   VDDQ   VSS   VDD
 F3   NC   NC   VSS   VDD   VREF
 F4   NC   VDDQ
 F5   NC   VDD
 F6   VSS   NC
 F7   NC   VDD
 F8   NC   VDDQ
 F9   NC   NC
 F10   NC   NC
 F11   VSS   VDDQ   VSS   VDD
 G1   NC   NC
 G2   NC   NC   VSS   VDD   VREF
 G3   VSS   VDDQ   VSS   VDD
 G4   NC   VDDQ
 G5   NC   VDD
 G6   VSS   NC
 G7   NC   VDD
 G8   NC   VDDQ
 G9   NC   NC
 G10   NC   NC
 G11   NC   NC   VSS   VDD   VREF
 H1   NC   NC   VSS   VDD   VREF
 H2   NC   VREF
 H3   NC   VDDQ
 H4   NC   VDDQ
 H5   NC   VDD
 H6   VSS   NC
 H7   NC   VDD
 H8   NC   VDDQ
 H9   NC   VDDQ
 H10   NC   VREF
 H11   NC   NC
 J1   NC   NC
 J2   NC   NC
 J3   NC   NC   VSS   VDD   VREF
 J4   NC   VDDQ
 J5   NC   VDD
 J6   VSS   NC
 J7   NC   VDD
 J8   NC   VDDQ
 J9   NC   NC
 J10   VSS   VDDQ   VSS   VDD
 J11   NC   NC   VSS   VDD   VREF
 K1   NC   NC
 K2   NC   NC
 K3   VSS   VDDQ   VSS   VDD
 K4   NC   VDDQ
 K5   NC   VDD
 K6   VSS   NC
 K7   NC   VDD
 K8   NC   VDDQ
 K9   NC   NC
 K10   NC   NC   VSS   VDD   VREF
 K11   VSS   VDDQ   VSS   VDD
 L1   NC   NC
 L2   VSS   VDDQ   VSS   VDD
 L3   NC   NC   VSS   VDD   VREF
 L4   NC   VDDQ
 L5   VSS   NC
 L6   VSS   NC
 L7   VSS   NC
 L8   NC   VDDQ
 L9   NC   NC
 L10   NC   NC
 L11   VSS   VDDQ   VSS   VDD
 M1   NC   NC
 M2   NC   NC
 M3   NC   NC   VSS   VDD   VREF
 M4   VSS   NC
 M5   VSS   NC
 M6   VSS   NC
 M7   VSS   NC
 M8   VSS   NC
 M9   NC   NC
 M10   VSS   VDDQ   VSS   VDD
 M11   NC   NC   VSS   VDD   VREF
 N1   NC   NC
 N2   NC   NC   VSS   VDD   VREF
 N3   VSS   VDDQ   VSS   VDD
 N4   VSS   NC
 N5   NC   NC   VSS   VDD   VREF
 N6   NC   NC   VSS   VDD   VREF
 N7   NC   NC   VSS   VDD   VREF
 N8   VSS   NC
 N9   NC   NC
 N10   NC   NC
 N11   NC   NC   VSS   VDD   VREF
 P1   NC   NC
 P2   NC   NC
 P3   VSS   VDDQ   VSS   VDD
 P4   NC   NC   VSS   VDD   VREF
 P5   NC   NC   VSS   VDD   VREF
 P6   VSS   VDDQ   VSS   VDD
 P7   NC   NC   VSS   VDD   VREF
 P8   NC   NC   VSS   VDD   VREF
 P9   NC   NC
 P10   NC   NC   VSS   VDD   VREF
 P11   VSS   VDDQ   VSS   VDD
 R1   VSS   VDDQ   VSS   VDD
 R2   NC   NC   VSS   VDD   VREF
 R3   NC   NC   VSS   VDD   VREF
 R4   NC   NC   VSS   VDD   VREF
 R5   NC   NC   VSS   VDD   VREF
 R6   NC   NC
 R7   NC   NC   VSS   VDD   VREF
 R8   NC   NC   VSS   VDD   VREF
 R9   NC   NC   VSS   VDD   VREF
 R10   NC   NC   VSS   VDD   VREF
 R11   NC   NC   VSS   VDD   VREF
[Pin]   signal_name model_name   R_pin   L_pin   C_pin
 A1   nCQ   ECHO   229m   1.82nH   0.656pF
 A2   SA   CONTROL   203m   1.74nH   0.634pF
 A3   SA   CONTROL   185m   1.59nH   0.518pF
 A4   nW   CONTROL   185m   1.38nH   0.583pF
 A5   nBW1   CONTROL   178m   1.36nH   0.540pF
 A6   nK   CONTROL   224m   1.64nH   0.652pF
 A7   NC   NC
 A8   nR   CONTROL   188m   1.49nH   0.551pF
 A9   SA   CONTROL   186m   1.48nH   0.595pF
 A10   SA   CONTROL   191m   1.70nH   0.568pF
 A11   CQ   ECHO   227m   1.84nH   0.605pF
 B1   NC   NC
 B2   Q9   PROGBUF   233m   1.94nH   0.666pF
 B3   D9   DIN   226m   2.49nH   0.560pF
 B4   SA   CONTROL   181m   1.49nH   0.521pF
 B5   NC   NC
 B6   K   CONTROL   221m   1.68nH   0.652pF
 B7   NBW0   CONTROL   178m   1.43nH   0.537pF
 B8   SA   CONTROL   181m   1.41nH   0.565pF
 B9   NC   NC
 B10   NC   NC
 B11   Q8   PROGBUF   232m   1.94nH   0.683pF
 C1   NC   NC
 C2   NC   NC
 C3   D10   DIN   241m   2.35nH   0.708pF
 C4   VSS   GND
 C5   SA   CONTROL   189m   1.61nH   0.614pF
 C6   NC   NC
 C7   SA   CONTROL   185m   1.72nH   0.535pF
 C8   VSS   GND
 C9   NC   NC
 C10   Q7   PROGBUF   231m   2.16nH   0.604pF
 C11   D8   DIN   219m   1.74nH   0.625pF
 D1   NC   NC
 D2   D11   DIN   227m   1.95nH   0.654pF
 D3   Q10   PROGBUF   256m   2.33nH   0.752pF
 D4   VSS   GND
 D5   VSS   GND
 D6   VSS   GND
 D7   VSS   GND
 D8   VSS   GND
 D9   NC   NC
 D10   NC   NC
 D11   D7   DIN   218m   1.75nH   0.605pF
 E1   NC   NC
 E2   NC   NC
 E3   Q11   PROGBUF   240m   2.04nH   0.712pF
 E4   VDDQ   POWER
 E5   VSS   GND
 E6   VSS   GND
 E7   VSS   GND
 E8   VDDQ   POWER
 E9   NC   NC
 E10   D6   DIN   223m   1.85nH   0.659pF
 E11   Q6   PROGBUF   225m   1.74nH   0.649pF
 F1   NC   NC
 F2   Q12   PROGBUF   230m   1.84nH   0.651pF
 F3   D12   DIN   230m   2.00nH   0.644pF
 F4   VDDQ   POWER
 F5   VDD   POWER
 F6   VSS   GND
 F7   VDD   POWER
 F8   VDDQ   POWER
 F9   NC   NC
 F10   NC   NC
 F11   Q5   PROGBUF   237m   1.82nH   0.690pF
 G1   NC   NC
 G2   D13   DIN   221m   1.73nH   0.669pF
 G3   Q13   PROGBUF   244m   2.11nH   0.723pF
 G4   VDDQ   POWER
 G5   VDD   POWER
 G6   VSS   GND
 G7   VDD   POWER
 G8   VDDQ   POWER
 G9   NC   NC
 G10   NC   NC
 G11   D5   DIN   217m   1.66nH   0.597pF
 H1   NDoff   CONTROL   254m   2.26nH   0.651pF
 H2   VREF   POWER
 H3   VDDQ   POWER
 H4   VDDQ   POWER
 H5   VDD   POWER
 H6   VSS   GND
 H7   VDD   POWER
 H8   VDDQ   POWER
 H9   VDDQ   POWER
 H10   VREF   POWER
 H11   ZQ   NC
 J1   NC   NC
 J2   NC   NC
 J3   D14   DIN   233m   2.02nH   0.708pF
 J4   VDDQ   POWER
 J5   VDD   POWER
 J6   VSS   GND
 J7   VDD   POWER
 J8   VDDQ   POWER
 J9   NC   NC
 J10   Q4   PROGBUF   231m   1.92nH   0.628pF
 J11   D4   DIN   222m   1.68nH   0.657pF
 K1   NC   NC
 K2   NC   NC
 K3   Q14   PROGBUF   238m   1.99nH   0.619pF
 K4   VDDQ   POWER
 K5   VDD   POWER
 K6   VSS   GND
 K7   VDD   POWER
 K8   VDDQ   POWER
 K9   NC   NC
 K10   D3   DIN   211m   1.71nH   0.543pF
 K11   Q3   PROGBUF   236m   1.79nH   0.629pF
 L1   NC   NC
 L2   Q15   PROGBUF   228m   1.89nH   0.672pF
 L3   D15   DIN   237m   2.14nH   0.663pF
 L4   VDDQ   POWER
 L5   VSS   GND
 L6   VSS   GND
 L7   VSS   GND
 L8   VDDQ   POWER
 L9   NC   NC
 L10   NC   NC
 L11   Q2   PROGBUF   223m   1.72nH   0.654pF
 M1   NC   NC
 M2   NC   NC
 M3   D16   DIN   246m   2.04nH   0.704pF
 M4   VSS   GND
 M5   VSS   GND
 M6   VSS   GND
 M7   VSS   GND
 M8   VSS   GND
 M9   NC   NC
 M10   Q1   PROGBUF   243m   2.05nH   0.690pF
 M11   D2   DIN   228m   1.90nH   0.609pF
 N1   NC   NC
 N2   D17   DIN   219m   1.88nH   0.569pF
 N3   Q16   PROGBUF   268m   2.36nH   0.730pF
 N4   VSS   GND
 N5   SA   CONTROL   186m   1.69nH   0.505pF
 N6   SA   CONTROL   191m   1.56nH   0.607pF
 N7   SA   CONTROL   193m   1.62nH   0.543pF
 N8   VSS   GND
 N9   NC   NC
 N10   NC   NC
 N11   D1   DIN   220m   1.66nH   0.645pF
 P1   NC   NC
 P2   NC   NC
 P3   Q17   PROGBUF   236m   2.33nH   0.676pF
 P4   SA   CONTROL   185m   1.52nH   0.546pF
 P5   SA   CONTROL   185m   1.41nH   0.604pF
 P6   QVLD   ECHO   184m   1.42nH   0.590pF
 P7   SA   CONTROL   192m   1.57nH   0.599pF
 P8   SA   CONTROL   195m   1.51nH   0.593pF
 P9   NC   NC
 P10   D0   DIN   221m   1.90nH   0.660pF
 P11   Q0   PROGBUF   236m   1.77nH   0.674pF
 R1   TDO   JTAG   151m   1.27nH   0.509pF
 R2   TCK   CONTROL   132m   1.10nH   0.478pF
 R3   SA   CONTROL   208m   1.92nH   0.490pF
 R4   SA   CONTROL   198m   1.58nH   0.599pF
 R5   SA   CONTROL   190m   1.46nH   0.609pF
 R6   NC   NC
 R7   SA   CONTROL   198m   1.47nH   0.632pF
 R8   SA   CONTROL   202m   1.49nH   0.640pF
 R9   SA   CONTROL   214m   1.68nH   0.647pF
 R10   TMS   CONTROL   148m   1.19nH   0.517pF
 R11   TDI   CONTROL   157m   1.27nH   0.525pF
[Component]   GS8662D20BD
[Manufacturer]   GSI Technology
[Package]
|  variable   typ   min   max
R_pkg   0.2   0.1   0.5
L_pkg   3nH   1nH   5nH
C_pkg   1.5pF   1pF   3pF
[Package Model]   8662xxxBD
[Pin Mapping] pulldown_ref pullup_ref gnd_clamp_ref power_clamp_ref ext_ref
|PIN   Pull-Down   Pull-Up   Power-clamp   Gnd-clamp   EXT-ref
 A1   VSS   VDDQ   VSS   VDD
 A2   NC   NC   VSS   VDD   VREF
 A3   NC   NC   VSS   VDD   VREF
 A4   NC   NC   VSS   VDD   VREF
 A5   NC   NC   VSS   VDD   VREF
 A6   NC   NC   VSS   VDD   VREF
 A7   NC   NC
 A8   NC   NC   VSS   VDD   VREF
 A9   NC   NC   VSS   VDD   VREF
 A10   NC   NC   VSS   VDD   VREF
 A11   VSS   VDDQ   VSS   VDD
 B1   NC   NC
 B2   VSS   VDDQ   VSS   VDD
 B3   NC   NC   VSS   VDD   VREF
 B4   NC   NC   VSS   VDD   VREF
 B5   NC   NC
 B6   NC   NC   VSS   VDD   VREF
 B7   NC   NC   VSS   VDD   VREF
 B8   NC   NC   VSS   VDD   VREF
 B9   NC   NC
 B10   NC   NC
 B11   VSS   VDDQ   VSS   VDD
 C1   NC   NC
 C2   NC   NC
 C3   NC   NC   VSS   VDD   VREF
 C4   VSS   NC
 C5   NC   NC   VSS   VDD   VREF
 C6   NC   NC
 C7   NC   NC   VSS   VDD   VREF
 C8   VSS   NC
 C9   NC   NC
 C10   VSS   VDDQ   VSS   VDD
 C11   NC   NC   VSS   VDD   VREF
 D1   NC   NC
 D2   NC   NC   VSS   VDD   VREF
 D3   VSS   VDDQ   VSS   VDD
 D4   VSS   NC
 D5   VSS   NC
 D6   VSS   NC
 D7   VSS   NC
 D8   VSS   NC
 D9   NC   NC
 D10   NC   NC
 D11   NC   NC   VSS   VDD   VREF
 E1   NC   NC
 E2   NC   NC
 E3   VSS   VDDQ   VSS   VDD
 E4   NC   VDDQ
 E5   VSS   NC
 E6   VSS   NC
 E7   VSS   NC
 E8   NC   VDDQ
 E9   NC   NC
 E10   NC   NC   VSS   VDD   VREF
 E11   VSS   VDDQ   VSS   VDD
 F1   NC   NC
 F2   VSS   VDDQ   VSS   VDD
 F3   NC   NC   VSS   VDD   VREF
 F4   NC   VDDQ
 F5   NC   VDD
 F6   VSS   NC
 F7   NC   VDD
 F8   NC   VDDQ
 F9   NC   NC
 F10   NC   NC
 F11   VSS   VDDQ   VSS   VDD
 G1   NC   NC
 G2   NC   NC   VSS   VDD   VREF
 G3   VSS   VDDQ   VSS   VDD
 G4   NC   VDDQ
 G5   NC   VDD
 G6   VSS   NC
 G7   NC   VDD
 G8   NC   VDDQ
 G9   NC   NC
 G10   NC   NC
 G11   NC   NC   VSS   VDD   VREF
 H1   NC   NC   VSS   VDD   VREF
 H2   NC   VREF
 H3   NC   VDDQ
 H4   NC   VDDQ
 H5   NC   VDD
 H6   VSS   NC
 H7   NC   VDD
 H8   NC   VDDQ
 H9   NC   VDDQ
 H10   NC   VREF
 H11   NC   NC
 J1   NC   NC
 J2   NC   NC
 J3   NC   NC   VSS   VDD   VREF
 J4   NC   VDDQ
 J5   NC   VDD
 J6   VSS   NC
 J7   NC   VDD
 J8   NC   VDDQ
 J9   NC   NC
 J10   VSS   VDDQ   VSS   VDD
 J11   NC   NC   VSS   VDD   VREF
 K1   NC   NC
 K2   NC   NC
 K3   VSS   VDDQ   VSS   VDD
 K4   NC   VDDQ
 K5   NC   VDD
 K6   VSS   NC
 K7   NC   VDD
 K8   NC   VDDQ
 K9   NC   NC
 K10   NC   NC   VSS   VDD   VREF
 K11   VSS   VDDQ   VSS   VDD
 L1   NC   NC
 L2   VSS   VDDQ   VSS   VDD
 L3   NC   NC   VSS   VDD   VREF
 L4   NC   VDDQ
 L5   VSS   NC
 L6   VSS   NC
 L7   VSS   NC
 L8   NC   VDDQ
 L9   NC   NC
 L10   NC   NC
 L11   VSS   VDDQ   VSS   VDD
 M1   NC   NC
 M2   NC   NC
 M3   NC   NC   VSS   VDD   VREF
 M4   VSS   NC
 M5   VSS   NC
 M6   VSS   NC
 M7   VSS   NC
 M8   VSS   NC
 M9   NC   NC
 M10   VSS   VDDQ   VSS   VDD
 M11   NC   NC   VSS   VDD   VREF
 N1   NC   NC
 N2   NC   NC   VSS   VDD   VREF
 N3   VSS   VDDQ   VSS   VDD
 N4   VSS   NC
 N5   NC   NC   VSS   VDD   VREF
 N6   NC   NC   VSS   VDD   VREF
 N7   NC   NC   VSS   VDD   VREF
 N8   VSS   NC
 N9   NC   NC
 N10   NC   NC
 N11   NC   NC   VSS   VDD   VREF
 P1   NC   NC
 P2   NC   NC
 P3   VSS   VDDQ   VSS   VDD
 P4   NC   NC   VSS   VDD   VREF
 P5   NC   NC   VSS   VDD   VREF
 P6   VSS   VDDQ   VSS   VDD
 P7   NC   NC   VSS   VDD   VREF
 P8   NC   NC   VSS   VDD   VREF
 P9   NC   NC
 P10   NC   NC   VSS   VDD   VREF
 P11   VSS   VDDQ   VSS   VDD
 R1   VSS   VDDQ   VSS   VDD
 R2   NC   NC   VSS   VDD   VREF
 R3   NC   NC   VSS   VDD   VREF
 R4   NC   NC   VSS   VDD   VREF
 R5   NC   NC   VSS   VDD   VREF
 R6   NC   NC
 R7   NC   NC   VSS   VDD   VREF
 R8   NC   NC   VSS   VDD   VREF
 R9   NC   NC   VSS   VDD   VREF
 R10   NC   NC   VSS   VDD   VREF
 R11   NC   NC   VSS   VDD   VREF
[Pin]   signal_name model_name   R_pin   L_pin   C_pin
 A1   nCQ   ECHO   229m   1.82nH   0.656pF
 A2   SA   CONTROL   203m   1.74nH   0.634pF
 A3   SA   CONTROL   185m   1.59nH   0.518pF
 A4   nW   CONTROL   185m   1.38nH   0.583pF
 A5   nBW1   CONTROL   178m   1.36nH   0.540pF
 A6   nK   CONTROL   224m   1.64nH   0.652pF
 A7   NC   NC
 A8   nR   CONTROL   188m   1.49nH   0.551pF
 A9   SA   CONTROL   186m   1.48nH   0.595pF
 A10   SA   CONTROL   191m   1.70nH   0.568pF
 A11   CQ   ECHO   227m   1.84nH   0.605pF
 B1   NC   NC
 B2   Q9   PROGBUF   233m   1.94nH   0.666pF
 B3   D9   DIN   226m   2.49nH   0.560pF
 B4   SA   CONTROL   181m   1.49nH   0.521pF
 B5   NC   NC
 B6   K   CONTROL   221m   1.68nH   0.652pF
 B7   NBW0   CONTROL   178m   1.43nH   0.537pF
 B8   SA   CONTROL   181m   1.41nH   0.565pF
 B9   NC   NC
 B10   NC   NC
 B11   Q8   PROGBUF   232m   1.94nH   0.683pF
 C1   NC   NC
 C2   NC   NC
 C3   D10   DIN   241m   2.35nH   0.708pF
 C4   VSS   GND
 C5   SA   CONTROL   189m   1.61nH   0.614pF
 C6   NC   NC
 C7   SA   CONTROL   185m   1.72nH   0.535pF
 C8   VSS   GND
 C9   NC   NC
 C10   Q7   PROGBUF   231m   2.16nH   0.604pF
 C11   D8   DIN   219m   1.74nH   0.625pF
 D1   NC   NC
 D2   D11   DIN   227m   1.95nH   0.654pF
 D3   Q10   PROGBUF   256m   2.33nH   0.752pF
 D4   VSS   GND
 D5   VSS   GND
 D6   VSS   GND
 D7   VSS   GND
 D8   VSS   GND
 D9   NC   NC
 D10   NC   NC
 D11   D7   DIN   218m   1.75nH   0.605pF
 E1   NC   NC
 E2   NC   NC
 E3   Q11   PROGBUF   240m   2.04nH   0.712pF
 E4   VDDQ   POWER
 E5   VSS   GND
 E6   VSS   GND
 E7   VSS   GND
 E8   VDDQ   POWER
 E9   NC   NC
 E10   D6   DIN   223m   1.85nH   0.659pF
 E11   Q6   PROGBUF   225m   1.74nH   0.649pF
 F1   NC   NC
 F2   Q12   PROGBUF   230m   1.84nH   0.651pF
 F3   D12   DIN   230m   2.00nH   0.644pF
 F4   VDDQ   POWER
 F5   VDD   POWER
 F6   VSS   GND
 F7   VDD   POWER
 F8   VDDQ   POWER
 F9   NC   NC
 F10   NC   NC
 F11   Q5   PROGBUF   237m   1.82nH   0.690pF
 G1   NC   NC
 G2   D13   DIN   221m   1.73nH   0.669pF
 G3   Q13   PROGBUF   244m   2.11nH   0.723pF
 G4   VDDQ   POWER
 G5   VDD   POWER
 G6   VSS   GND
 G7   VDD   POWER
 G8   VDDQ   POWER
 G9   NC   NC
 G10   NC   NC
 G11   D5   DIN   217m   1.66nH   0.597pF
 H1   NDoff   CONTROL   254m   2.26nH   0.651pF
 H2   VREF   POWER
 H3   VDDQ   POWER
 H4   VDDQ   POWER
 H5   VDD   POWER
 H6   VSS   GND
 H7   VDD   POWER
 H8   VDDQ   POWER
 H9   VDDQ   POWER
 H10   VREF   POWER
 H11   ZQ   NC
 J1   NC   NC
 J2   NC   NC
 J3   D14   DIN   233m   2.02nH   0.708pF
 J4   VDDQ   POWER
 J5   VDD   POWER
 J6   VSS   GND
 J7   VDD   POWER
 J8   VDDQ   POWER
 J9   NC   NC
 J10   Q4   PROGBUF   231m   1.92nH   0.628pF
 J11   D4   DIN   222m   1.68nH   0.657pF
 K1   NC   NC
 K2   NC   NC
 K3   Q14   PROGBUF   238m   1.99nH   0.619pF
 K4   VDDQ   POWER
 K5   VDD   POWER
 K6   VSS   GND
 K7   VDD   POWER
 K8   VDDQ   POWER
 K9   NC   NC
 K10   D3   DIN   211m   1.71nH   0.543pF
 K11   Q3   PROGBUF   236m   1.79nH   0.629pF
 L1   NC   NC
 L2   Q15   PROGBUF   228m   1.89nH   0.672pF
 L3   D15   DIN   237m   2.14nH   0.663pF
 L4   VDDQ   POWER
 L5   VSS   GND
 L6   VSS   GND
 L7   VSS   GND
 L8   VDDQ   POWER
 L9   NC   NC
 L10   NC   NC
 L11   Q2   PROGBUF   223m   1.72nH   0.654pF
 M1   NC   NC
 M2   NC   NC
 M3   D16   DIN   246m   2.04nH   0.704pF
 M4   VSS   GND
 M5   VSS   GND
 M6   VSS   GND
 M7   VSS   GND
 M8   VSS   GND
 M9   NC   NC
 M10   Q1   PROGBUF   243m   2.05nH   0.690pF
 M11   D2   DIN   228m   1.90nH   0.609pF
 N1   NC   NC
 N2   D17   DIN   219m   1.88nH   0.569pF
 N3   Q16   PROGBUF   268m   2.36nH   0.730pF
 N4   VSS   GND
 N5   SA   CONTROL   186m   1.69nH   0.505pF
 N6   SA   CONTROL   191m   1.56nH   0.607pF
 N7   SA   CONTROL   193m   1.62nH   0.543pF
 N8   VSS   GND
 N9   NC   NC
 N10   NC   NC
 N11   D1   DIN   220m   1.66nH   0.645pF
 P1   NC   NC
 P2   NC   NC
 P3   Q17   PROGBUF   236m   2.33nH   0.676pF
 P4   SA   CONTROL   185m   1.52nH   0.546pF
 P5   SA   CONTROL   185m   1.41nH   0.604pF
 P6   QVLD   ECHO   184m   1.42nH   0.590pF
 P7   SA   CONTROL   192m   1.57nH   0.599pF
 P8   SA   CONTROL   195m   1.51nH   0.593pF
 P9   NC   NC
 P10   D0   DIN   221m   1.90nH   0.660pF
 P11   Q0   PROGBUF   236m   1.77nH   0.674pF
 R1   TDO   JTAG   151m   1.27nH   0.509pF
 R2   TCK   CONTROL   132m   1.10nH   0.478pF
 R3   SA   CONTROL   208m   1.92nH   0.490pF
 R4   SA   CONTROL   198m   1.58nH   0.599pF
 R5   SA   CONTROL   190m   1.46nH   0.609pF
 R6   NC   NC
 R7   SA   CONTROL   198m   1.47nH   0.632pF
 R8   SA   CONTROL   202m   1.49nH   0.640pF
 R9   SA   CONTROL   214m   1.68nH   0.647pF
 R10   TMS   CONTROL   148m   1.19nH   0.517pF
 R11   TDI   CONTROL   157m   1.27nH   0.525pF
[Component]   GS8662D36BD
[Manufacturer]   GSI Technology
[Package]
|  variable   typ   min   max
R_pkg   0.2   0.1   0.5
L_pkg   3nH   1nH   5nH
C_pkg   1.5pF   1pF   3pF
[Package Model]   8662xxxBD
[Pin Mapping] pulldown_ref pullup_ref gnd_clamp_ref power_clamp_ref ext_ref
|PIN   Pull-Down   Pull-Up   Power-clamp   Gnd-clamp   EXT-ref
 A1   VSS   VDDQ   VSS   VDD
 A2   NC   NC
 A3   NC   NC   VSS   VDD   VREF
 A4   NC   NC   VSS   VDD   VREF
 A5   NC   NC   VSS   VDD   VREF
 A6   NC   NC   VSS   VDD   VREF
 A7   NC   NC   VSS   VDD   VREF
 A8   NC   NC   VSS   VDD   VREF
 A9   NC   NC   VSS   VDD   VREF
 A10   NC   NC   VSS   VDD   VREF
 A11   VSS   VDDQ   VSS   VDD
 B1   VSS   VDDQ   VSS   VDD
 B2   VSS   VDDQ   VSS   VDD
 B3   NC   NC   VSS   VDD   VREF
 B4   NC   NC   VSS   VDD   VREF
 B5   NC   NC   VSS   VDD   VREF
 B6   NC   NC   VSS   VDD   VREF
 B7   NC   NC   VSS   VDD   VREF
 B8   NC   NC   VSS   VDD   VREF
 B9   NC   NC   VSS   VDD   VREF
 B10   VSS   VDDQ   VSS   VDD
 B11   VSS   VDDQ   VSS   VDD
 C1   NC   NC   VSS   VDD   VREF
 C2   VSS   VDDQ   VSS   VDD
 C3   NC   NC   VSS   VDD   VREF
 C4   VSS   NC
 C5   NC   NC   VSS   VDD   VREF
 C6   NC   NC
 C7   NC   NC   VSS   VDD   VREF
 C8   VSS   NC
 C9   NC   NC   VSS   VDD   VREF
 C10   VSS   VDDQ   VSS   VDD
 C11   NC   NC   VSS   VDD   VREF
 D1   NC   NC   VSS   VDD   VREF
 D2   NC   NC   VSS   VDD   VREF
 D3   VSS   VDDQ   VSS   VDD
 D4   VSS   NC
 D5   VSS   NC
 D6   VSS   NC
 D7   VSS   NC
 D8   VSS   NC
 D9   VSS   VDDQ   VSS   VDD
 D10   NC   NC   VSS   VDD   VREF
 D11   NC   NC   VSS   VDD   VREF
 E1   VSS   VDDQ   VSS   VDD
 E2   NC   NC   VSS   VDD   VREF
 E3   VSS   VDDQ   VSS   VDD
 E4   NC   VDDQ
 E5   VSS   NC
 E6   VSS   NC
 E7   VSS   NC
 E8   NC   VDDQ
 E9   VSS   VDDQ   VSS   VDD
 E10   NC   NC   VSS   VDD   VREF
 E11   VSS   VDDQ   VSS   VDD
 F1   VSS   VDDQ   VSS   VDD
 F2   VSS   VDDQ   VSS   VDD
 F3   NC   NC   VSS   VDD   VREF
 F4   NC   VDDQ
 F5   NC   VDD
 F6   VSS   NC
 F7   NC   VDD
 F8   NC   VDDQ
 F9   NC   NC   VSS   VDD   VREF
 F10   VSS   VDDQ   VSS   VDD
 F11   VSS   VDDQ   VSS   VDD
 G1   NC   NC   VSS   VDD   VREF
 G2   NC   NC   VSS   VDD   VREF
 G3   VSS   VDDQ   VSS   VDD
 G4   NC   VDDQ
 G5   NC   VDD
 G6   VSS   NC
 G7   NC   VDD
 G8   NC   VDDQ
 G9   VSS   VDDQ   VSS   VDD
 G10   NC   NC   VSS   VDD   VREF
 G11   NC   NC   VSS   VDD   VREF
 H1   NC   NC   VSS   VDD   VREF
 H2   NC   VREF
 H3   NC   VDDQ
 H4   NC   VDDQ
 H5   NC   VDD
 H6   VSS   NC
 H7   NC   VDD
 H8   NC   VDDQ
 H9   NC   VDDQ
 H10   NC   VREF
 H11   NC   NC
 J1   NC   NC   VSS   VDD   VREF
 J2   VSS   VDDQ   VSS   VDD
 J3   NC   NC   VSS   VDD   VREF
 J4   NC   VDDQ
 J5   NC   VDD
 J6   VSS   NC
 J7   NC   VDD
 J8   NC   VDDQ
 J9   NC   NC   VSS   VDD   VREF
 J10   VSS   VDDQ   VSS   VDD
 J11   NC   NC   VSS   VDD   VREF
 K1   VSS   VDDQ   VSS   VDD
 K2   NC   NC   VSS   VDD   VREF
 K3   VSS   VDDQ   VSS   VDD
 K4   NC   VDDQ
 K5   NC   VDD
 K6   VSS   NC
 K7   NC   VDD
 K8   NC   VDDQ
 K9   VSS   VDDQ   VSS   VDD
 K10   NC   NC   VSS   VDD   VREF
 K11   VSS   VDDQ   VSS   VDD
 L1   VSS   VDDQ   VSS   VDD
 L2   VSS   VDDQ   VSS   VDD
 L3   NC   NC   VSS   VDD   VREF
 L4   NC   VDDQ
 L5   VSS   NC
 L6   VSS   NC
 L7   VSS   NC
 L8   NC   VDDQ
 L9   NC   NC   VSS   VDD   VREF
 L10   VSS   VDDQ   VSS   VDD
 L11   VSS   VDDQ   VSS   VDD
 M1   NC   NC   VSS   VDD   VREF
 M2   VSS   VDDQ   VSS   VDD
 M3   NC   NC   VSS   VDD   VREF
 M4   VSS   NC
 M5   VSS   NC
 M6   VSS   NC
 M7   VSS   NC
 M8   VSS   NC
 M9   NC   NC   VSS   VDD   VREF
 M10   VSS   VDDQ   VSS   VDD
 M11   NC   NC   VSS   VDD   VREF
 N1   NC   NC   VSS   VDD   VREF
 N2   NC   NC   VSS   VDD   VREF
 N3   VSS   VDDQ   VSS   VDD
 N4   VSS   NC
 N5   NC   NC   VSS   VDD   VREF
 N6   NC   NC   VSS   VDD   VREF
 N7   NC   NC   VSS   VDD   VREF
 N8   VSS   NC
 N9   VSS   VDDQ   VSS   VDD
 N10   NC   NC   VSS   VDD   VREF
 N11   NC   NC   VSS   VDD   VREF
 P1   VSS   VDDQ   VSS   VDD
 P2   NC   NC   VSS   VDD   VREF
 P3   VSS   VDDQ   VSS   VDD
 P4   NC   NC   VSS   VDD   VREF
 P5   NC   NC   VSS   VDD   VREF
 P6   NC   NC   VSS   VDD   VREF
 P7   NC   NC   VSS   VDD   VREF
 P8   NC   NC   VSS   VDD   VREF
 P9   VSS   VDDQ   VSS   VDD
 P10   NC   NC   VSS   VDD   VREF
 P11   VSS   VDDQ   VSS   VDD
 R1   VSS   VDDQ   VSS   VDD
 R2   NC   NC   VSS   VDD   VREF
 R3   NC   NC   VSS   VDD   VREF
 R4   NC   NC   VSS   VDD   VREF
 R5   NC   NC   VSS   VDD   VREF
 R6   NC   NC   VSS   VDD   VREF
 R7   NC   NC   VSS   VDD   VREF
 R8   NC   NC   VSS   VDD   VREF
 R9   NC   NC   VSS   VDD   VREF
 R10   NC   NC   VSS   VDD   VREF
 R11   NC   NC   VSS   VDD   VREF
[Pin]   signal_name model_name   R_pin   L_pin   C_pin
 A1   nCQ   ECHO   229m   1.82nH   0.656pF
 A2   NC   NC
 A3   SA   CONTROL   185m   1.59nH   0.518pF
 A4   nW   CONTROL   185m   1.38nH   0.583pF
 A5   nBW2   CONTROL   178m   1.36nH   0.540pF
 A6   nK   CONTROL   224m   1.64nH   0.652pF
 A7   nBW1   CONTROL   185m   1.39nH   0.547pF
 A8   nR   CONTROL   188m   1.49nH   0.551pF
 A9   SA   CONTROL   186m   1.48nH   0.595pF
 A10   SA   CONTROL   191m   1.70nH   0.568pF
 A11   CQ   ECHO   227m   1.84nH   0.605pF
 B1   Q27   PROGBUF   233m   1.94nH   0.668pF
 B2   Q18   PROGBUF   233m   1.94nH   0.666pF
 B3   D18   DIN   226m   2.49nH   0.560pF
 B4   SA   CONTROL   181m   1.49nH   0.521pF
 B5   nBW3   CONTROL   183m   1.40nH   0.575pF
 B6   K   CONTROL   221m   1.68nH   0.652pF
 B7   NBW0   CONTROL   178m   1.43nH   0.537pF
 B8   SA   CONTROL   181m   1.41nH   0.565pF
 B9   D17   DIN   223m   2.31nH   0.578pF
 B10   Q17   PROGBUF   229m   1.99nH   0.652pF
 B11   Q8   PROGBUF   232m   1.94nH   0.683pF
 C1   D27   DIN   224m   1.71nH   0.644pF
 C2   Q28   PROGBUF   240m   2.04nH   0.699pF
 C3   D19   DIN   241m   2.35nH   0.708pF
 C4   VSS   GND
 C5   SA   CONTROL   189m   1.61nH   0.614pF
 C6   NC   NC
 C7   SA   CONTROL   185m   1.72nH   0.535pF
 C8   VSS   GND
 C9   D16   DIN   226m   2.17nH   0.581pF
 C10   Q7   PROGBUF   231m   2.16nH   0.604pF
 C11   D8   DIN   219m   1.74nH   0.625pF
 D1   D28   DIN   216m   1.82nH   0.523pF
 D2   D20   DIN   227m   1.95nH   0.654pF
 D3   Q19   PROGBUF   256m   2.33nH   0.752pF
 D4   VSS   GND
 D5   VSS   GND
 D6   VSS   GND
 D7   VSS   GND
 D8   VSS   GND
 D9   Q16   PROGBUF   252m   2.26nH   0.751pF
 D10   D15   DIN   224m   2.00nH   0.622pF
 D11   D7   DIN   218m   1.75nH   0.605pF
 E1   Q29   PROGBUF   226m   1.75nH   0.668pF
 E2   D29   DIN   220m   1.79nH   0.660pF
 E3   Q20   PROGBUF   240m   2.04nH   0.712pF
 E4   VDDQ   POWER
 E5   VSS   GND
 E6   VSS   GND
 E7   VSS   GND
 E8   VDDQ   POWER
 E9   Q15   PROGBUF   243m   2.04nH   0.712pF
 E10   D6   DIN   223m   1.85nH   0.659pF
 E11   Q6   PROGBUF   225m   1.74nH   0.649pF
 F1   Q30   PROGBUF   238m   1.87nH   0.672pF
 F2   Q21   PROGBUF   230m   1.84nH   0.651pF
 F3   D21   DIN   230m   2.00nH   0.644pF
 F4   VDDQ   POWER
 F5   VDD   POWER
 F6   VSS   GND
 F7   VDD   POWER
 F8   VDDQ   POWER
 F9   D14   DIN   234m   1.97nH   0.703pF
 F10   Q14   PROGBUF   234m   1.83nH   0.660pF
 F11   Q5   PROGBUF   237m   1.82nH   0.690pF
 G1   D30   DIN   218m   1.67nH   0.641pF
 G2   D22   DIN   221m   1.73nH   0.669pF
 G3   Q22   PROGBUF   244m   2.11nH   0.723pF
 G4   VDDQ   POWER
 G5   VDD   POWER
 G6   VSS   GND
 G7   VDD   POWER
 G8   VDDQ   POWER
 G9   Q13   PROGBUF   238m   1.88nH   0.707pF
 G10   D13   DIN   218m   1.76nH   0.576pF
 G11   D5   DIN   217m   1.66nH   0.597pF
 H1   NDoff   CONTROL   254m   2.26nH   0.651pF
 H2   VREF   POWER
 H3   VDDQ   POWER
 H4   VDDQ   POWER
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| Models and submodels in the file (23): VIO_18_50 (I/O), VIO_15_50 (I/O), VIO_18_35 (I/O), VIO_15_35 (I/O), VIO_18_50_ODT (I/O), VIO_15_50_ODT (I/O), VIO_18_35_ODT (I/O), VIO_15_35_ODT (I/O), VOUT_18_50 (Output), VOUT_15_50 (Output), VOUT_18_35 (Output), VOUT_15_35 (Output), JTAG (Output), VCQ_18_50 (Output), VCQ_15_50 (Output), VCQ_18_35 (Output), VCQ_15_35 (Output), CONTROL_18 (Input), CONTROL_15 (Input), DIN_18 (Input), DIN_15 (Input), Strong_ODT_18V (Dynamic_clamp), Strong_ODT_15V (Dynamic_clamp)
